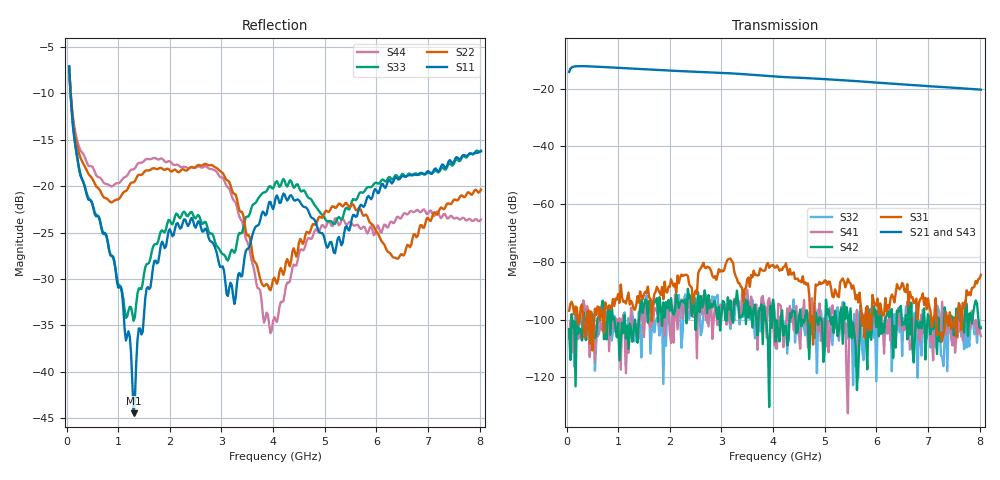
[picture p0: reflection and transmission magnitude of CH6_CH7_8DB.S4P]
!Agilent Technologies,E5071C,MY46316741,A.11.02
!Date: Mon Jun 01 10:34:37 2026
!Data & Calibration Information:
!1:CH6 INPUT 2:CH6 OUTPUT 3:CH7 INPUT 4:CH7 OUTPUT
!Freq	S11:SOLT4(ON)	S12:SOLT4(ON)	S13:SOLT4(ON)	S14:SOLT4(ON)
!	S21:SOLT4(ON)	S22:SOLT4(ON)	S23:SOLT4(ON)	S24:SOLT4(ON)
!	S31:SOLT4(ON)	S32:SOLT4(ON)	S33:SOLT4(ON)	S34:SOLT4(ON)
!	S41:SOLT4(ON)	S42:SOLT4(ON)	S43:SOLT4(ON)	S44:SOLT4(ON)
!PortZ  Port1:50+j0  Port2:50+j0  Port3:50+j0  Port4:50+j0
!Above PortZ is port z conversion or system Z0 setting when saving the data.
!When reading, reference impedance value at option line is always used.
# Hz S dB R 50
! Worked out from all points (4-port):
!   320 points, 50 MHz to 8.025 GHz, reference 50 ohm
!   strongest paths, dB at 50 MHz, 2.05 GHz, 4.05 GHz, 6.05 GHz, 8.025 GHz:
!     S21: -14.3, -13.8, -15.9, -18.0, -20.4
!     S43: -14.2, -13.8, -15.9, -18.0, -20.4
!     S31: -96.9, -87.3, -82.0, -98.3, -84.5
!     S42: -103.3, -97.7, -107.7, -105.8, -102.9
!     S41: -106.5, -98.1, -100.0, -97.0, -105.8
!     S32: -105.1, -100.3, -109.9, -97.6, -102.5
!   lowest |S11| = -44.5 dB at 1.3 GHz (marker M1), VSWR 1.01, Z = 49.5 - j0.313 ohm
!   |S11| at or under -10 dB: 78.35 MHz to end of sweep
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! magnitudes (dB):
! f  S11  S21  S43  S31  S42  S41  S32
! 50 MHz  -7.1  -14.3  -14.2  -96.9  -103.3  -106.5  -105.1
! 1.3 GHz  -44.5  -13.2  -13.2  -96.4  -104.0  -101.2  -103.5
! 2.125 GHz  -24.1  -13.9  -13.8  -90.7  -91.2  -96.6  -97.1
! 3.25 GHz  -32.7  -14.8  -14.8  -83.5  -93.3  -92.8  -100.3
! 3.95 GHz  -21.7  -15.7  -15.8  -81.3  -95.2  -96.1  -94.0
! 5.075 GHz  -26.4  -16.8  -16.8  -86.8  -96.5  -111.3  -97.5
! 8.025 GHz  -16.3  -20.4  -20.4  -84.5  -102.9  -105.8  -102.5
